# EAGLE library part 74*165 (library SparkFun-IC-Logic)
8-Bit Shift Register (Parallel to Serial) Datasheet SparkFun Products SparkFun Shift-In Breakout - SN74HC165 (BOB-11733)
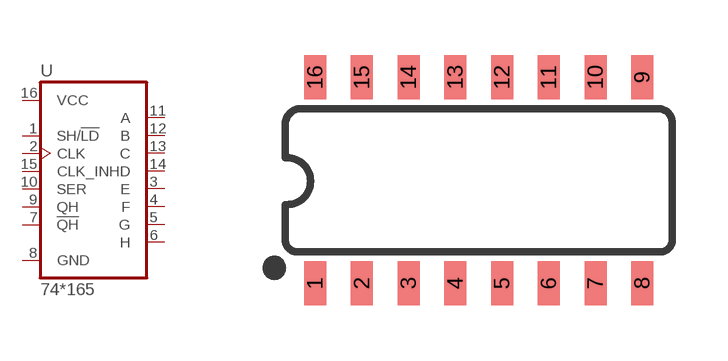
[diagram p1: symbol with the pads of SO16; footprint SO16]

Designator prefix U

## 74HC165D (PROD_ID: IC-11325; VALUE: SN74HC165DR)  [SO16]
1  SH/!LD  in
2  CLK  in
3  E  hiz
4  F  hiz
5  G  hiz
6  H  hiz
7  !QH  in
8  GND  pwr
9  QH  hiz
10  SER  in
11  A  hiz
12  B  hiz
13  C  hiz
14  D  hiz
15  CLK_INH  in
16  VCC  pwr

## Footprint SO16 (pad centres in mm)
SOIC, 0.15 inch width
smd 0.6 x 1.2: 1 -4.445,-2.8; 2 -3.175,-2.8; 3 -1.905,-2.8; 4 -0.635,-2.8; 5 0.635,-2.8; 6 1.905,-2.8; 7 3.175,-2.8; 8 4.445,-2.8; 9 4.445,2.8; 10 3.175,2.8; 11 1.905,2.8; 12 0.635,2.8; 13 -0.635,2.8; 14 -1.905,2.8; 15 -3.175,2.8; 16 -4.445,2.8

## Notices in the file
Licensing: Creative Commons ShareAlike 4.0 International - https://creativecommons.org/licenses/by-sa/4.0
